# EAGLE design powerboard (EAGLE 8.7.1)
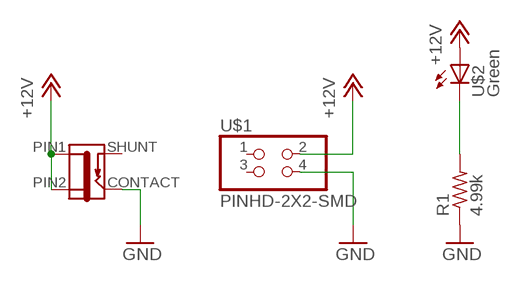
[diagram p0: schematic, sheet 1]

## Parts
J1  JACK-2.1MM  [PJ-002AH-SMT]
R1  4.99k  RES-US1206FAB  [R1206FAB]
U$1  PINHD-2X2-SMD  [2X02SMD]
U$2  Green  LEDFAB1206  [LED1206FAB]

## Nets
+12V: J1.PIN1 J1.PIN2 U$1.2 U$2.1(A)
GND: J1.CONTACT R1.1 U$1.4
N$1: R1.2 U$2.2(C)
Unconnected: U$1.1 U$1.3

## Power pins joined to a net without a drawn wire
SHUNT: J1.SHUNT

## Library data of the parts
J1 = fab:JACK-2.1MM: SMD DC power jack PJ-002AH-SMT As found in the fablab inventory. Made by Zaerc.
R1 = fab:RES-US: Resistor (US Symbol)
U$1 = fab:PINHD-2X2-SMD
U$2 = fab:LED: LED

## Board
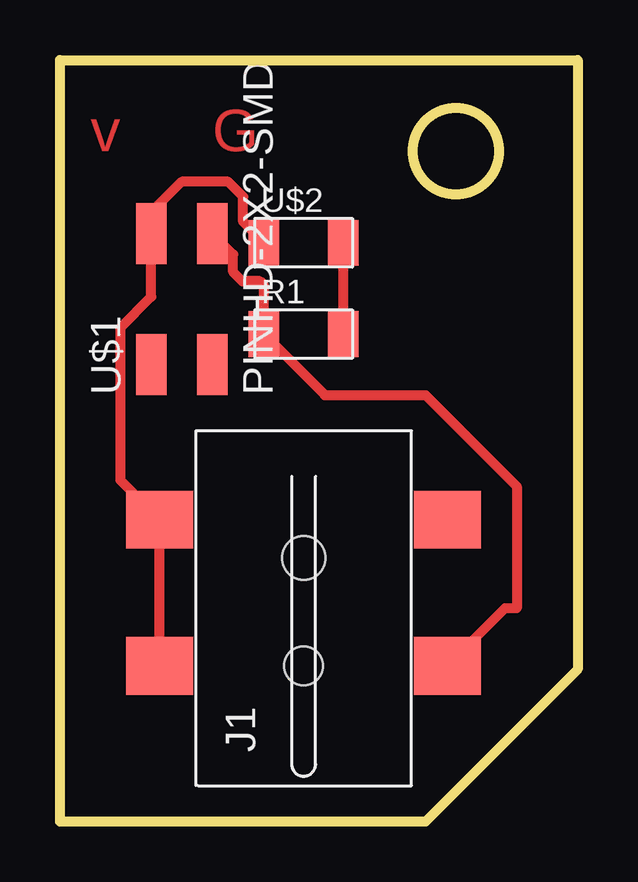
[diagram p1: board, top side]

Size 21.59 x 31.75 mm. Coordinates in mm from the lower left corner, seen from the top.
Outline: 0,31.42 0,0
Outline: 0,0 0,31.75 21.59,31.75 21.59,6.35 15.24,0 0,0
Outline: circle at 16.51,27.94 radius 1.8
Copper layers 1: Top 0.035mm
Design rules "basbasic": minimum track width 0.3mm, minimum drill 0.9mm, track to track 0.45mm, track to pad 0.45mm, pad to pad 0.45mm, via to via 0.45mm, smd to smd 6mil, copper to edge 40mil, drill to drill 6mil, minimum pad ring 10mil, minimum via ring 8mil, stop-mask expansion 4mil, vias tented up to drill 0mil, thermal gap 10mil

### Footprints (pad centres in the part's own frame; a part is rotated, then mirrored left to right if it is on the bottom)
PJ-002AH-SMT = smd 2.4 x 2.8: CONTACT -2.4,-6; PIN1 3.7,6; PIN2 -2.4,6; SHUNT 3.7,-6 | hole 1.6: -2.4,0 | hole 1.8: 2.1,0
R1206FAB = smd 1.27 x 1.905: 1 -1.651,0; 2 1.651,0
2X02SMD = smd 2.54 x 1.27: 1 -2.54,1.27; 2 2.92,1.27; 3 -2.54,-1.27; 4 2.92,-1.27
LED1206FAB = smd 1.27 x 1.905: 1 -1.651,0; 2 1.651,0

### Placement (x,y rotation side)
J1  10.16,8.89 90 top
R1  10.16,20.32 0 top
U$1  5.08,21.59 90 top
U$2  10.16,24.13 0 top

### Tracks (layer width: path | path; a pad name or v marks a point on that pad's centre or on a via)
+12V
  Top 0.406: J1.PIN2 J1.PIN1 2.52,14.23 2.52,20.59 3.81,21.88 U$1.2 3.81,25.4 5.08,26.67 7.02,26.67 7.64,26.05 7.64,25 U$2.1
GND
  Top 0.406: J1.CONTACT 18.56,8.89 19.05,8.89 19.05,13.97 15.24,17.78 11.05,17.78 R1.1 8.51,22.35 8.34,22.52 7.6,22.52 7.22,22.91 7.22,23.64 U$1.4
N$1
  Top 0.406: U$2.2 R1.2

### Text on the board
Top: v | G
